DATA_BLOCK DB 102
TITLE =BLOCK DATA FOR ALARM PRESS TD_17 AND OP_37
AUTHOR : Esposito
FAMILY : EGAL_srl
NAME : BL_DATA
VERSION : 0.1


  STRUCT
   Al_auxiliary_OFF : BOOL ;	//Alarm auxiliary OFF
   Al_safety_jack : BOOL ;	//Alarm safety jacks fault
   Al_emer_stop_OCP : BOOL ;	//Alarm emergency stop on control pannel
   Al_emer_stop_OFRU : BOOL ;	//Alarm emergency stop on front right upright
   Al_emer_stop_ORRU : BOOL ;	//Alarm emergency stop on rear right upright
   Al_emer_stop_OFLU : BOOL ;	//Alarm emergency stop on front left upright
   Al_emer_stop_ORLU : BOOL ;	//Alarm emergency stop on rear left upright
   Al_emer_stop_OPC : BOOL ;	//Alarm emergency stop on press cabinet
   Al_battery_PLC : BOOL ;	//Alarm battery PLC system
   Al_CPU_active : BOOL ;	//Alarm CPU active
   Al_modul_FM352 : BOOL ;	//Alarm module FM352 active
   Al_modul_SM338 : BOOL ;	//Alarm module SM338 active
   Al_modul_analog : BOOL ;	//Alarm module analogical PLC
   Al_modul_digit : BOOL ;	//Alarm module digital PLC
   DB102_1_6 : BOOL ;
   DB102_1_7 : BOOL ;
   Al_count_part : BOOL ;	//Alarm counter partial full
   Al_count_main : BOOL ;	//Alarm counter totaly full
   Al_Hands_dev : BOOL ;	//Alarm two hands device
   Al_cir_stop : BOOL ;	//Alarm circuit cycle stop device
   Al_clamp_unlock : BOOL ;	//Alarm clamps circuit front and rear not unlock
   DB102_DBX2_5 : BOOL ;
   Al_clamps_Pressure : BOOL ;	//Alarm low pressure lock clamps circuit
   Al_clamps_lock : BOOL ;	//Alarm clamps circuit front and rear not lock
   Al_emer_stop_SMOL : BOOL ;	//Alarm emergency stop safety module or line
   DB102_DBX3_1 : BOOL ;
   DB102_DBX3_2 : BOOL ;
   Al_checks_rotation : BOOL ;	//Alarm breakdown check rotation
   Al_rot_reliaf : BOOL ;	//Alarm rotation not relief
   Al_dead_point : BOOL ;	//Alarm press not upper dead point
   Al_sel_slide : BOOL ;	//Alarm selector switch enable slide adjustment
   Al_sel_overload : BOOL ;	//Alarm selector switch enable overload
   Al_Hi_oil_overload : BOOL ;	//Alarm hight oil level overload
   Al_Hi_pre_overload : BOOL ;	//Alarm hight overload pressure
   Al_Lo_pre_overload : BOOL ;	//Alarm low overload pressure
   Al_Lo_pre_balanc : BOOL ;	//Alarm low balancing pressure
   Al_TH_PSAM : BOOL ;	//Alarm thermal protection slide adjustment motor
   Al_slide_AMI : BOOL ;	//Alarm slide adjustment motor inverter
   DB102_DB4_6 : BOOL ;
   DB102_DB4_7 : BOOL ;
   DB102_DBX5_0 : BOOL ;
   Al_TH_PPL : BOOL ;	//Alarm thermal protection pump lubrication
   Al_CC_PL : BOOL ;	//Alarm clogged contactor pump lubrication
   Al_BMAC_PL : BOOL ;	//Alarm been missing answer contactor pump lubrication
   Al_LL_OL : BOOL ;	//Alarm low level oil lubrication
   Al_LP_CL : BOOL ;	//Alarm low pressure circuit lubrication
   Al_LM_tabon : BOOL ;	//Alarm lubrication monitor trabon
   Al_LL_OO : BOOL ;	//Alarm low oil level overload
   Al_LP_FWC : BOOL ;	//Alarm low pressure fly wheel circuit
   Al_TH_PPTP : BOOL ;	//Alarm thermal protection pump torc pac
   Al_BMAC_PTP : BOOL ;	//Alarm been missing answer contactor pump torc pac
   Al_CC_PTP : BOOL ;	//Alarm clogged contactor pump torc pac
   Al_TH_TPCF : BOOL ;	//Alarm thermal protection torc pac cooling fan
   Al_BMAC_TPCF : BOOL ;	//Alarm been missing answer contactor torc pac cooling fan
   Al_CC_TPCF : BOOL ;	//Alarm clogged contactor torc pac cooling fan
   Al_LL_OTP : BOOL ;	//Alarm oil low level torc pac
   Al_TH_SAM : BOOL ;	//Alarm temperature hight slide adjustment motor
   Al_TH_maim_MS : BOOL ;	//Alarm temperature hight main motor supply
   Al_TH_PMM : BOOL ;	//Alarm thermal protection main motor
   Al_C_main_M : BOOL ;	//Alarm converter main motor
   Al_LC_main_M : BOOL ;	//Alarm line contactor main motor
   Al_speed_MM : BOOL ;	//Alarm speed main motor
   Al_field_EF : BOOL ;	//Alarm field enable fault
   Al_C_EF : BOOL ;	//Alarm converter enable fault
   DB102_DBX8_0 : BOOL ;
   DB102_DBX8_1 : BOOL ;
   DB102_DBX8_2 : BOOL ;
   DB102_DBX8_3 : BOOL ;
   DB102_DBX8_4 : BOOL ;
   DB102_DBX8_5 : BOOL ;
   DB102_DBX8_6 : BOOL ;
   DB102_DBX8_7 : BOOL ;
   Al_HT_OTP : BOOL ;	//Alarm oil high temperature torc pac
   Al_LP_oil_TPLT : BOOL ;	//Alarm oil low pressure torc pac lubrication tank
   Al_LP_oil_CTPLT : BOOL ;	//Alarm oil pressure cooling torc pac lubrication tank
   Al_Double_SC : BOOL ;	//Alarm double stroke control
   Al_clutch_UCNO : BOOL ;	//Alarm clucth brake unit control not ok
   Al_clutch_BPNO : BOOL ;	//Alarm clutch brake pressure not OK
   DB102_DBX9_6 : BOOL ;
   DB102_DBX9_7 : BOOL ;
   Al_TH_PIORRU : BOOL ;	//Alarm thermal protection inlet one rear right upright
   Al_TH_PITRRU : BOOL ;	//Alarm thermal protection inlet two rear right upright
   Al_BMCA_IORRU : BOOL ;	//Alarm been missing contactor answer inlet one rear right upright
   Al_BMCA_ITRRU : BOOL ;	//Alarm been missing contactor answer inlet two rear right upright
   Al_CC_IORRU : BOOL ;	//Alarm clogged contactor inlet one rear right upright
   Al_CC_ITRRU : BOOL ;	//Alarm clogged contactor inlet two rear right upright
   DB102_DBX10_6 : BOOL ;
   DB102_DBX10_7 : BOOL ;
   Al_scrap_FARNO : BOOL ;	//Alarm scrapes cutes front and rear not open
   Al_scrap_FARNC : BOOL ;	//Alarm scrapes cutes front and rear not close
   Al_TH_PIOFRU : BOOL ;	//Alarm thermal protection inlet one front right upright
   Al_TH_PITFRU : BOOL ;	//Alarm thermal protection inlet two front right upright
   Al_BMCA_IOFRU : BOOL ;	//Alarm been missing contactor answer inlet one fornt right upright
   Al_CC_IOFRU : BOOL ;	//Alarm clogged contactor inlet one front right upright
   Al_BMCA_ITFRU : BOOL ;	//Alarm been missing contactor answer inlet two fornt right upright
   Al_CC_ITFRU : BOOL ;	//Alarm clogged contactor answer inlet two front right upright
   Al_periph_09 : BOOL ;	//Alarm gate 1 not closed and locked
   Al_periph_0A : BOOL ;	//Alarm gate 2 not closed and locked
   Al_periph_0B : BOOL ;	//Alarm gate 3 not closed and locked
   Al_periph_0C : BOOL ;	//Alarm gate 4 not closed and locked
   Al_periph_0D : BOOL ;	//Alarm gate 5 not closed and locked
   Al_periph_0E : BOOL ;	//Alarm gate 6 not closed and locked
   Al_periph_0F : BOOL ;	//Alarm gate 7 not closed and locked
   Al_periph_10 : BOOL ;	//Alarm lightcurtain blankcarts
   Al_periph_01 : BOOL ;	//Alarm emergency stop operator panel blankcarts
   Al_periph_02 : BOOL ;	//Alarm emergency stop gate blankcart1
   Al_periph_03 : BOOL ;	//Alarm emergency stop gate blankcart2
   Al_periph_04 : BOOL ;	//Alarm emergency stop auxiliary robot cabinet 1
   Al_periph_05 : BOOL ;	//Alarm emergency stop auxiliary robot cabinet 2
   Al_periph_06 : BOOL ;	//Alarm emergency stop gate robot 1
   Al_periph_07 : BOOL ;	//Alarm emergency stop gate robot 2
   Al_periph_08 : BOOL ;	//Alarm emergency stop handterminal centering table
   Al_conv_CCR : BOOL ;	//Alarm current control relay conveyor
   Al_conv_MP : BOOL ;	//Alarm motor protection coveyor
   Al_conv_FPS : BOOL ;	//Alarm fault proximity switch
   Al_conv_ML : BOOL ;	//Alarm minimum level lubrication conveyor
   Al_conv_ES : BOOL ;	//Alarm emergency stop conveyor
   DBX : BOOL ;
   DBX1 : BOOL ;
   DBX2 : BOOL ;
   Al_periph_11 : BOOL ;	//Alarm overload motors auxiliary equipment
   Al_periph_12 : BOOL ;	//Alarm powersupply auxiliary equipment
   Al_periph_13 : BOOL ;	//Alarm overload powersupply operatorpanel blankcarts
   DBX3 : BOOL ;
   DBX4 : BOOL ;
   DBX5 : BOOL ;
   DBX6 : BOOL ;
   DBX7 : BOOL ;
   DBX8 : BOOL ;
   DBX9 : BOOL ;
   DBX10 : BOOL ;
   DBX11 : BOOL ;
   DBX12 : BOOL ;
   DBX13 : BOOL ;
   DBX14 : BOOL ;
   DBX15 : BOOL ;
   DBX16 : BOOL ;
   DBX17 : BOOL ;
   DBX18 : BOOL ;
   DBX19 : BOOL ;
   DBX20 : BOOL ;
   DBX21 : BOOL ;
   DBX22 : BOOL ;
   DBX23 : BOOL ;
   DBX24 : BOOL ;
   DBX25 : BOOL ;
   DBX26 : BOOL ;
   DBX27 : BOOL ;
   DBX28 : BOOL ;
   DBX29 : BOOL ;
   DBX30 : BOOL ;
   DBX31 : BOOL ;
   DBX32 : BOOL ;
   DBX33 : BOOL ;
   DBX34 : BOOL ;
   DBX35 : BOOL ;
   DBX36 : BOOL ;
   DBX37 : BOOL ;
   DBX38 : BOOL ;
   DBX39 : BOOL ;
   DBX40 : BOOL ;
   DBX41 : BOOL ;
   DBX42 : BOOL ;
   DBX43 : BOOL ;
   DBX44 : BOOL ;
   DBX45 : BOOL ;
   DBX46 : BOOL ;
   DBX47 : BOOL ;
   DBX48 : BOOL ;
   DBX49 : BOOL ;
   DBX50 : BOOL ;
   DBX51 : BOOL ;
   DBX52 : BOOL ;
   DBX53 : BOOL ;
   DBX54 : BOOL ;
   DBX55 : BOOL ;
   DBX56 : BOOL ;
   DBX57 : BOOL ;
   DBX58 : BOOL ;
   DBX59 : BOOL ;
   DBX60 : BOOL ;
   DBX61 : BOOL ;
   DBX62 : BOOL ;
   DBX63 : BOOL ;
   DBX64 : BOOL ;
   DBX65 : BOOL ;
   DBX66 : BOOL ;
   DBX67 : BOOL ;
   DBX68 : BOOL ;
   DBX69 : BOOL ;
   DBX70 : BOOL ;
   DBX71 : BOOL ;
   DBX72 : BOOL ;
   DBX73 : BOOL ;
   DBX74 : BOOL ;
   DBX75 : BOOL ;
   DBX76 : BOOL ;
   DBX77 : BOOL ;
   DBX78 : BOOL ;
   DBX79 : BOOL ;
   DBX80 : BOOL ;
   DBX81 : BOOL ;
   DBX82 : BOOL ;
   DBX83 : BOOL ;
   DBX84 : BOOL ;
   DBX85 : BOOL ;
   DBX86 : BOOL ;
   DBX87 : BOOL ;
   DBX88 : BOOL ;
   DBX89 : BOOL ;
   DBX90 : BOOL ;
   DBX91 : BOOL ;
   DBX92 : BOOL ;
   DBX93 : BOOL ;
   DBX94 : BOOL ;
   DBX95 : BOOL ;
   DBX96 : BOOL ;
   DBX97 : BOOL ;
   DBX98 : BOOL ;
   DBX99 : BOOL ;
   DBX100 : BOOL ;
   DBX101 : BOOL ;
   DBX102 : BOOL ;
   DBX103 : BOOL ;
   DBX104 : BOOL ;
   DBX105 : BOOL ;
   DBX106 : BOOL ;
   DBX107 : BOOL ;
   DBX108 : BOOL ;
   DBX109 : BOOL ;
   DBX110 : BOOL ;
   DBX111 : BOOL ;
   DBX112 : BOOL ;
   DBX113 : BOOL ;
   DBX114 : BOOL ;
   DBX115 : BOOL ;
   DBX116 : BOOL ;
   DBX117 : BOOL ;
   DBX118 : BOOL ;
   DBX119 : BOOL ;
   Al_rot_encoder : BOOL ;	//Alarm for fault rotation Encoder press
   DBX121 : BOOL ;
   DBX122 : BOOL ;
   DBX123 : BOOL ;
   DBX124 : BOOL ;
   DBX125 : BOOL ;
   DBX126 : BOOL ;
   DBX127 : BOOL ;
   DBX128 : BOOL ;
   DBX129 : BOOL ;
   DBX130 : BOOL ;
   DBX131 : BOOL ;
   DBX132 : BOOL ;
   DBX133 : BOOL ;
   DBX134 : BOOL ;
   DBX135 : BOOL ;
  END_STRUCT ;
BEGIN
   Al_auxiliary_OFF := FALSE;
   Al_safety_jack := FALSE;
   Al_emer_stop_OCP := FALSE;
   Al_emer_stop_OFRU := FALSE;
   Al_emer_stop_ORRU := FALSE;
   Al_emer_stop_OFLU := FALSE;
   Al_emer_stop_ORLU := FALSE;
   Al_emer_stop_OPC := FALSE;
   Al_battery_PLC := FALSE;
   Al_CPU_active := FALSE;
   Al_modul_FM352 := FALSE;
   Al_modul_SM338 := FALSE;
   Al_modul_analog := FALSE;
   Al_modul_digit := FALSE;
   DB102_1_6 := FALSE;
   DB102_1_7 := FALSE;
   Al_count_part := FALSE;
   Al_count_main := FALSE;
   Al_Hands_dev := FALSE;
   Al_cir_stop := FALSE;
   Al_clamp_unlock := FALSE;
   DB102_DBX2_5 := FALSE;
   Al_clamps_Pressure := FALSE;
   Al_clamps_lock := FALSE;
   Al_emer_stop_SMOL := FALSE;
   DB102_DBX3_1 := FALSE;
   DB102_DBX3_2 := FALSE;
   Al_checks_rotation := FALSE;
   Al_rot_reliaf := FALSE;
   Al_dead_point := FALSE;
   Al_sel_slide := FALSE;
   Al_sel_overload := FALSE;
   Al_Hi_oil_overload := FALSE;
   Al_Hi_pre_overload := FALSE;
   Al_Lo_pre_overload := FALSE;
   Al_Lo_pre_balanc := FALSE;
   Al_TH_PSAM := FALSE;
   Al_slide_AMI := FALSE;
   DB102_DB4_6 := FALSE;
   DB102_DB4_7 := FALSE;
   DB102_DBX5_0 := FALSE;
   Al_TH_PPL := FALSE;
   Al_CC_PL := FALSE;
   Al_BMAC_PL := FALSE;
   Al_LL_OL := FALSE;
   Al_LP_CL := FALSE;
   Al_LM_tabon := FALSE;
   Al_LL_OO := FALSE;
   Al_LP_FWC := FALSE;
   Al_TH_PPTP := FALSE;
   Al_BMAC_PTP := FALSE;
   Al_CC_PTP := FALSE;
   Al_TH_TPCF := FALSE;
   Al_BMAC_TPCF := FALSE;
   Al_CC_TPCF := FALSE;
   Al_LL_OTP := FALSE;
   Al_TH_SAM := FALSE;
   Al_TH_maim_MS := FALSE;
   Al_TH_PMM := FALSE;
   Al_C_main_M := FALSE;
   Al_LC_main_M := FALSE;
   Al_speed_MM := FALSE;
   Al_field_EF := FALSE;
   Al_C_EF := FALSE;
   DB102_DBX8_0 := FALSE;
   DB102_DBX8_1 := FALSE;
   DB102_DBX8_2 := FALSE;
   DB102_DBX8_3 := FALSE;
   DB102_DBX8_4 := FALSE;
   DB102_DBX8_5 := FALSE;
   DB102_DBX8_6 := FALSE;
   DB102_DBX8_7 := FALSE;
   Al_HT_OTP := FALSE;
   Al_LP_oil_TPLT := FALSE;
   Al_LP_oil_CTPLT := FALSE;
   Al_Double_SC := FALSE;
   Al_clutch_UCNO := FALSE;
   Al_clutch_BPNO := FALSE;
   DB102_DBX9_6 := FALSE;
   DB102_DBX9_7 := FALSE;
   Al_TH_PIORRU := FALSE;
   Al_TH_PITRRU := FALSE;
   Al_BMCA_IORRU := FALSE;
   Al_BMCA_ITRRU := FALSE;
   Al_CC_IORRU := FALSE;
   Al_CC_ITRRU := FALSE;
   DB102_DBX10_6 := FALSE;
   DB102_DBX10_7 := FALSE;
   Al_scrap_FARNO := FALSE;
   Al_scrap_FARNC := FALSE;
   Al_TH_PIOFRU := FALSE;
   Al_TH_PITFRU := FALSE;
   Al_BMCA_IOFRU := FALSE;
   Al_CC_IOFRU := FALSE;
   Al_BMCA_ITFRU := FALSE;
   Al_CC_ITFRU := FALSE;
   Al_periph_09 := FALSE;
   Al_periph_0A := FALSE;
   Al_periph_0B := FALSE;
   Al_periph_0C := FALSE;
   Al_periph_0D := FALSE;
   Al_periph_0E := FALSE;
   Al_periph_0F := FALSE;
   Al_periph_10 := FALSE;
   Al_periph_01 := FALSE;
   Al_periph_02 := FALSE;
   Al_periph_03 := FALSE;
   Al_periph_04 := FALSE;
   Al_periph_05 := FALSE;
   Al_periph_06 := FALSE;
   Al_periph_07 := FALSE;
   Al_periph_08 := FALSE;
   Al_conv_CCR := FALSE;
   Al_conv_MP := FALSE;
   Al_conv_FPS := FALSE;
   Al_conv_ML := FALSE;
   Al_conv_ES := FALSE;
   DBX := FALSE;
   DBX1 := FALSE;
   DBX2 := FALSE;
   Al_periph_11 := FALSE;
   Al_periph_12 := FALSE;
   Al_periph_13 := FALSE;
   DBX3 := FALSE;
   DBX4 := FALSE;
   DBX5 := FALSE;
   DBX6 := FALSE;
   DBX7 := FALSE;
   DBX8 := FALSE;
   DBX9 := FALSE;
   DBX10 := FALSE;
   DBX11 := FALSE;
   DBX12 := FALSE;
   DBX13 := FALSE;
   DBX14 := FALSE;
   DBX15 := FALSE;
   DBX16 := FALSE;
   DBX17 := FALSE;
   DBX18 := FALSE;
   DBX19 := FALSE;
   DBX20 := FALSE;
   DBX21 := FALSE;
   DBX22 := FALSE;
   DBX23 := FALSE;
   DBX24 := FALSE;
   DBX25 := FALSE;
   DBX26 := FALSE;
   DBX27 := FALSE;
   DBX28 := FALSE;
   DBX29 := FALSE;
   DBX30 := FALSE;
   DBX31 := FALSE;
   DBX32 := FALSE;
   DBX33 := FALSE;
   DBX34 := FALSE;
   DBX35 := FALSE;
   DBX36 := FALSE;
   DBX37 := FALSE;
   DBX38 := FALSE;
   DBX39 := FALSE;
   DBX40 := FALSE;
   DBX41 := FALSE;
   DBX42 := FALSE;
   DBX43 := FALSE;
   DBX44 := FALSE;
   DBX45 := FALSE;
   DBX46 := FALSE;
   DBX47 := FALSE;
   DBX48 := FALSE;
   DBX49 := FALSE;
   DBX50 := FALSE;
   DBX51 := FALSE;
   DBX52 := FALSE;
   DBX53 := FALSE;
   DBX54 := FALSE;
   DBX55 := FALSE;
   DBX56 := FALSE;
   DBX57 := FALSE;
   DBX58 := FALSE;
   DBX59 := FALSE;
   DBX60 := FALSE;
   DBX61 := FALSE;
   DBX62 := FALSE;
   DBX63 := FALSE;
   DBX64 := FALSE;
   DBX65 := FALSE;
   DBX66 := FALSE;
   DBX67 := FALSE;
   DBX68 := FALSE;
   DBX69 := FALSE;
   DBX70 := FALSE;
   DBX71 := FALSE;
   DBX72 := FALSE;
   DBX73 := FALSE;
   DBX74 := FALSE;
   DBX75 := FALSE;
   DBX76 := FALSE;
   DBX77 := FALSE;
   DBX78 := FALSE;
   DBX79 := FALSE;
   DBX80 := FALSE;
   DBX81 := FALSE;
   DBX82 := FALSE;
   DBX83 := FALSE;
   DBX84 := FALSE;
   DBX85 := FALSE;
   DBX86 := FALSE;
   DBX87 := FALSE;
   DBX88 := FALSE;
   DBX89 := FALSE;
   DBX90 := FALSE;
   DBX91 := FALSE;
   DBX92 := FALSE;
   DBX93 := FALSE;
   DBX94 := FALSE;
   DBX95 := FALSE;
   DBX96 := FALSE;
   DBX97 := FALSE;
   DBX98 := FALSE;
   DBX99 := FALSE;
   DBX100 := FALSE;
   DBX101 := FALSE;
   DBX102 := FALSE;
   DBX103 := FALSE;
   DBX104 := FALSE;
   DBX105 := FALSE;
   DBX106 := FALSE;
   DBX107 := FALSE;
   DBX108 := FALSE;
   DBX109 := FALSE;
   DBX110 := FALSE;
   DBX111 := FALSE;
   DBX112 := FALSE;
   DBX113 := FALSE;
   DBX114 := FALSE;
   DBX115 := FALSE;
   DBX116 := FALSE;
   DBX117 := FALSE;
   DBX118 := FALSE;
   DBX119 := FALSE;
   Al_rot_encoder := FALSE;
   DBX121 := FALSE;
   DBX122 := FALSE;
   DBX123 := FALSE;
   DBX124 := FALSE;
   DBX125 := FALSE;
   DBX126 := FALSE;
   DBX127 := FALSE;
   DBX128 := FALSE;
   DBX129 := FALSE;
   DBX130 := FALSE;
   DBX131 := FALSE;
   DBX132 := FALSE;
   DBX133 := FALSE;
   DBX134 := FALSE;
   DBX135 := FALSE;
END_DATA_BLOCK

